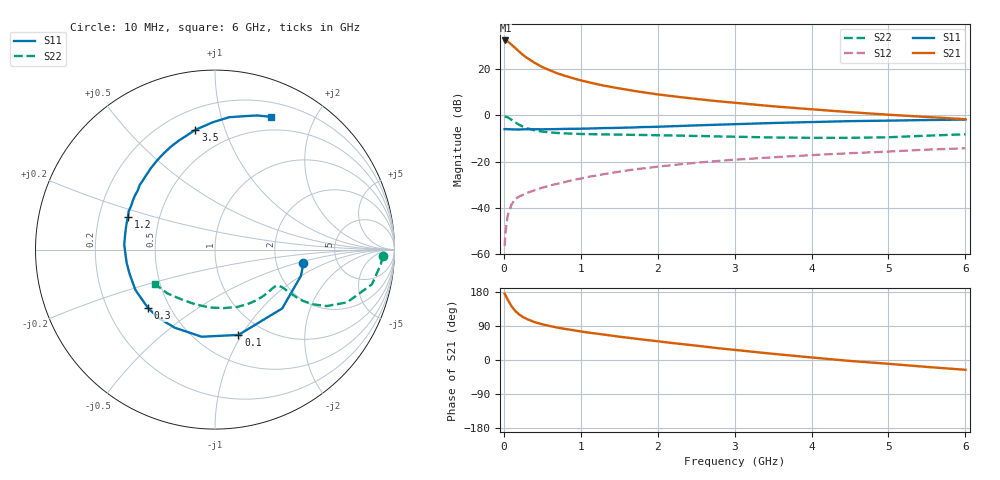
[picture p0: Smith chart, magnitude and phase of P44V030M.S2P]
! SIEMENS Small Signal Semiconductors
! BFP182
! Si NPN RF Bipolar Junction Transistor in SOT143
! VCE = 4 V  IC = 30 mA
! Common Emitter S-Parameters:  March  1996
# GHz  S  MA  R  50
!  f  S11  S21  S12  S22
! GHz  MAG  ANG  MAG  ANG  MAG  ANG  MAG  ANG
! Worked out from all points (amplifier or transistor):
!   36 points, 10 MHz to 6 GHz, reference 50 ohm
!   highest |S21| = 32.2 dB at 20 MHz (marker M1)
!   |S21| within 3 dB of that: start of sweep to 139.6 MHz
!   unconditionally stable (mu >= 1): 543.9 MHz to 5.554 GHz
!   at 250 MHz: K = 0.64, MSG = 30.1 dB, |S12| = -34.3 dB
!   at 1.4 GHz: K = 1.26, MAG = 15.4 dB, |S12| = -24.9 dB
!   at 6 GHz: K = 0.96, MSG = 6.3 dB, |S12| = -14.3 dB
!   S11 on the Smith chart (normalised r, x): 10 MHz: 2.86, -0.55; 100 MHz: 0.77, -0.97; 300 MHz: 0.38, -0.33; 1.2 GHz: 0.33, +0.16; 3.5 GHz: 0.32, +0.80; 6 GHz: 0.35, +1.45
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0.01  0.4983 -8.4  40.63 175.4  0.0015 76.6  0.9347 -2.2
0.02  0.5008 -17.0  40.63 171.5  0.0028 79.3  0.9282 -4.9
0.05  0.4976 -41.2  38.73 159.1  0.0068 75.3  0.8954 -12.5
0.1  0.493 -74.6  33.03 141.9  0.0119 61.7  0.7922 -21.8
0.15  0.4911 -98.7  27.73 129.3  0.0156 56.8  0.6955 -26.9
0.2  0.4892 -117.0  23.32 120.0  0.0177 54.0  0.6193 -29.4
0.25  0.4944 -129.5  19.75 113.2  0.0192 51.3  0.5628 -30.3
0.3  0.495 -139.0  17.15 108.1  0.0211 51.8  0.5218 -30.3
0.4  0.4972 -153.1  13.41 100.0  0.024 52.8  0.4715 -29.9
0.5  0.4946 -163.8  10.86 94.2  0.0273 52.6  0.4414 -29.4
0.6  0.4976 -171.1  9.199 89.5  0.0304 55.4  0.4234 -29.3
0.7  0.5002 -177.8  7.889 85.4  0.0333 56.8  0.4119 -29.5
0.8  0.5063 176.9  6.999 81.8  0.0364 56.9  0.4034 -30.0
1.1  0.5142 163.0  5.121 72.3  0.0468 57.6  0.3893 -32.8
1.2  0.5186 159.2  4.685 69.8  0.0499 57.6  0.3865 -34.0
1.7  0.5422 142.5  3.307 56.6  0.068 55.7  0.3752 -41.7
2.2  0.5765 128.6  2.548 44.6  0.0841 52.1  0.3642 -51.0
2.8  0.623 113.4  1.978 30.8  0.1032 46.8  0.3468 -64.0
3.5  0.6763 99.3  1.55 16.3  0.1234 40.7  0.3296 -81.6
4.5  0.7418 83.9  1.158 -2.5  0.1511 31.9  0.3241 -109.9
5.5  0.7832 72.6  0.913 -18.3  0.1807 23.4  0.3605 -137.4
6  0.8034 67.0  0.817 -25.8  0.1928 18.3  0.3859 -150.3
